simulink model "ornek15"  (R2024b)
settings: Solver=VariableStepAuto  StartTime=0.0  StopTime=20  RelTol=1e-3

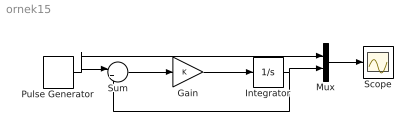
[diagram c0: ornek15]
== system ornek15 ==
  Gain : Gain
  Integrator : Integrator
  Mux : Mux  Inputs=2
  Pulse Generator : DiscretePulseGenerator  PulseType=Time based  Amplitude=12  Period=10  PulseWidth=50
  Scope : Scope
  Sum : Sum  Inputs=|+-
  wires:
  Pulse Generator/1 -> Mux/1, Sum/1
  Sum/1 -> Gain/1
  Gain/1 -> Integrator/1
  Integrator/1 -> Sum/2, Mux/2
  Mux/1 -> Scope/1
